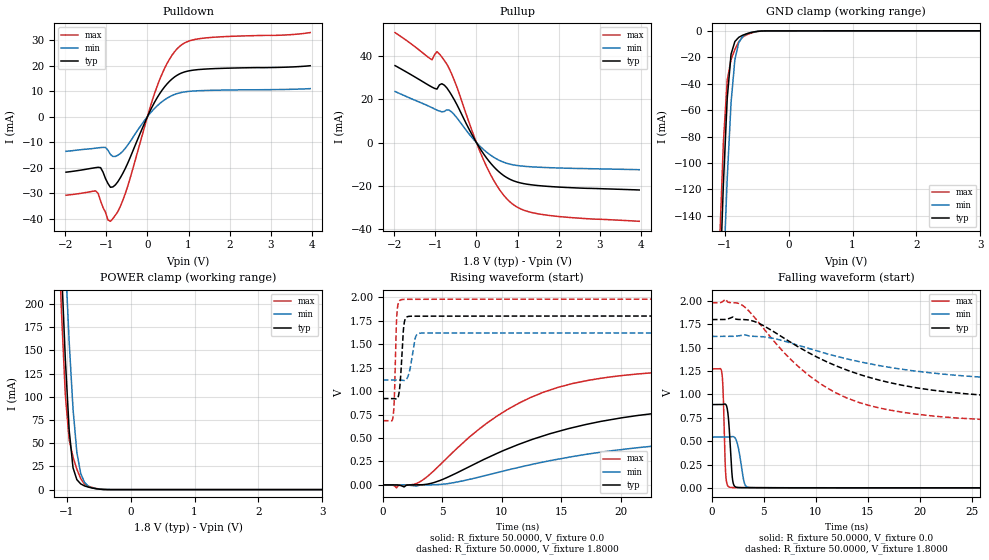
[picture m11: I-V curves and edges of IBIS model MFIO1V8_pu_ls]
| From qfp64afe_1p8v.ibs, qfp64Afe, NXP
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[Model] MFIO1V8_pu_ls
|   Model MFIO1V8_pu_ls
| This model was characterised for following simulation conditions:
| External (pad) voltage:
|   - Typ: 1.8V,   - Min: 1.62V,   - Max: 1.98V
| Library cells for typ/min/max conditions are connected as defined below:
|  IO - External Pad
|  A - Core Input
|  EN - Output Buffer Enable
|  BOOST - vdde
|  EHS - gnd
|  ENZI - vdd
|  EPD - gnd
|  EPUN - gnd
|  ZI - NC
|  ZIF - NC
|  gnd - gnd
|  gnde - gnde
|  vdd - vdd
|  vdde - vdde
| All other pins connected to ground
Model_type I/O
Polarity   Non-Inverting
Enable   Active-Low
Vinl =   0.5400V
Vinh =   1.2600V
Vmeas =  0.9000V
Cref =   0.0F
Rref =   100.0000
Vref =   0.0V
C_comp   1.5959pF   1.5126pF   1.6704pF
|C_comp_pullup   0.7872pF   0.8189pF   0.7436pF
|C_comp_pulldown   0.5957pF   0.6344pF   0.5599pF
[Model Spec]
| variable   typ   min   max
Vinh   0.5400V   0.4860V   0.5940V
Vinl   1.2600V   1.1340V   1.3860V
Vmeas   0.9000V   0.8100V   0.9900V
[Temperature Range]   25.0000   0.1250k   -40.0000
[Voltage Range]   1.8000V   1.6200V   1.9800V
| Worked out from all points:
|   slope of the pulldown table from 0 to 0.27 V, typ, clamps not added: 32.6 ohm
|   slope of the pullup table from 0 to 0.27 V, typ, clamps not added: 34.8 ohm
|   GND clamp passes 1 mA (typ) near -0.56 V on its own axis
|   POWER clamp passes 1 mA (typ) near -0.54 V on its own axis
|   rising waveform, R_fixture 50.0000, V_fixture 0.0: 20-80 % time 12.9ns typ, 15.7ns min, 9.09ns max; typ from 0.001 V to 0.891 V
|   rising waveform, R_fixture 50.0000, V_fixture 1.8000: 20-80 % time 250ps typ, 393ps min, 168ps max; typ from 0.921 V to 1.8 V
|   falling waveform, R_fixture 50.0000, V_fixture 0.0: 20-80 % time 296ps typ, 476ps min, 197ps max; typ from 0.891 V to 0.001 V
|   falling waveform, R_fixture 50.0000, V_fixture 1.8000: 20-80 % time 11.7ns typ, 13.6ns min, 8.56ns max; typ from 1.8 V to 0.921 V
[Pulldown]
|Voltage   I(typ)   I(min)   I(max)
-1.98V    -21.74mA   -13.58mA   -30.76mA
-1.26V    -19.96mA   -12.33mA   -29.04mA
-1.14V    -19.96mA   -12.1mA    -33mA
-960mV    -26.19mA   -13.15mA   -40.44mA
-840mV    -27.51mA   -15.58mA   -39.92mA
-540mV    -20.34mA   -12.41mA   -30.2mA
60mV      2.086mA    1.197mA    3.341mA
300mV     9.043mA    5.145mA    14.58mA
540mV     13.88mA    7.813mA    22.59mA
840mV     17.16mA    9.517mA    28.23mA
1.44V     18.67mA    10.27mA    30.87mA
3.96V     19.95mA    10.98mA    32.93mA
[Pullup]
|Voltage   I(typ)   I(min)   I(max)
-1.98V    35.7mA     23.68mA    51.03mA
-1.08V    25.71mA    16.17mA    38.42mA
-960mV    24.81mA    15.04mA    42.18mA
-840mV    27.29mA    14.27mA    39.65mA
-720mV    25.36mA    15.21mA    36.42mA
-540mV    19.88mA    12.94mA    28.95mA
-60mV     2.002mA    1.263mA    3.041mA
240mV     -7.02mA    -4.333mA   -10.88mA
600mV     -14.41mA   -8.644mA   -22.88mA
900mV     -17.74mA   -10.36mA   -28.83mA
1.74V     -20.33mA   -11.62mA   -33.75mA
3.96V     -22mA      -12.58mA   -36.53mA
[GND_clamp]
|Voltage   I(typ)   I(min)   I(max)
-1.98V    -1.781A    -1.801A    -1.77A
-1.08V    -200.2mA   -270.3mA   -162.2mA
-1.02V    -116mA     -186.3mA   -84.54mA
-960mV    -51.3mA    -111.9mA   -37.4mA
-900mV    -17.69mA   -54.47mA   -21.74mA
-840mV    -8.055mA   -21.72mA   -14.12mA
-780mV    -4.959mA   -8.992mA   -8.359mA
-720mV    -3.374mA   -4.47mA    -4.799mA
-600mV    -1.439mA   -1.366mA   -1.942mA
-480mV    -366uA     -375.1uA   -469.4uA
-360mV    -62.42uA   -67.25uA   -76.06uA
3.96V     0A         0A         0A
[POWER_clamp]
|Voltage   I(typ)   I(min)   I(max)
-1.98V    2.119A     2.147A     2.105A
-1.14V    349.2mA    450mA      300.5mA
-1.08V    239.1mA    345.9mA    191.2mA
-1.02V    140.4mA    247.8mA    101.6mA
-960mV    64.04mA    159.3mA    53.84mA
-900mV    23.56mA    87.21mA    35.07mA
-840mV    10.75mA    40.17mA    22.03mA
-780mV    6.182mA    17.48mA    11.88mA
-720mV    3.977mA    7.724mA    5.963mA
-600mV    1.704mA    1.818mA    2.322mA
-360mV    31.78uA    68.22uA    27.15uA
3.96V     0A         0A         0A
[Ramp]
| variable   typ   min   max
dV/dt_r  0.5342/12.9472n   0.3254/15.7052n   0.7632/9.0881n
dV/dt_f  0.5274/11.7431n   0.3009/13.6080n   0.7767/8.5548n
R_load = 50.0000
[Rising Waveform]
R_fixture= 50.0000
V_fixture= 0.0
V_fixture_min= 0.0
V_fixture_max= 0.0
|time   V(typ)   V(min)   V(max)
0s        636.5uV    684uV      594.3uV
1.143ns   588.1uV    702uV      -30.91mV
3.203ns   1.63mV     -537.3uV   39.42mV
4.956ns   55.11mV    6.837mV    232.7mV
8.014ns   241.9mV    81.4mV     587.6mV
12.33ns   474.1mV    212.9mV    926.3mV
15.97ns   611.4mV    303mV      1.081V
21.24ns   736.7mV    394.5mV    1.18V
40.28ns   869.7mV    518mV      1.262V
100ns     890.9mV    543.1mV    1.273V
[Rising Waveform]
R_fixture= 50.0000
V_fixture= 1.8000
V_fixture_min= 1.6200
V_fixture_max= 1.9800
|time   V(typ)   V(min)   V(max)
0s        920.9mV    1.118V     685.4mV
847.9ps   921.1mV    1.118V     718.1mV
969.6ps   919.2mV    1.119V     934.2mV
1.204ns   918.4mV    1.119V     1.857V
1.441ns   1.063V     1.117V     1.968V
1.682ns   1.563V     1.114V     1.977V
1.952ns   1.783V     1.121V     1.978V
2.739ns   1.798V     1.572V     1.978V
3.266ns   1.798V     1.618V     1.978V
100ns     1.8V       1.62V      1.98V
[Falling Waveform]
R_fixture= 50.0000
V_fixture= 0.0
V_fixture_min= 0.0
V_fixture_max= 0.0
|time   V(typ)   V(min)   V(max)
0s        891mV      543.2mV    1.273V
954.2ps   891.2mV    543.2mV    1.237V
1.08ns    893.2mV    543.2mV    1.041V
1.347ns   891.4mV    543mV      127mV
1.579ns   763.2mV    544mV      15.76mV
1.811ns   371.8mV    547.1mV    5.267mV
2.131ns   27.06mV    545.1mV    3.544mV
3.155ns   2.666mV    43.29mV    3.519mV
3.779ns   2.782mV    2.922mV    2.864mV
100ns     636.6uV    684.1uV    594.3uV
[Falling Waveform]
R_fixture= 50.0000
V_fixture= 1.8000
V_fixture_min= 1.6200
V_fixture_max= 1.9800
|time   V(typ)   V(min)   V(max)
0s        1.8V       1.62V      1.98V
1.307ns   1.801V     1.62V      2.019V
3.054ns   1.8V       1.635V     1.944V
4.714ns   1.75V      1.618V     1.741V
7.87ns    1.538V     1.54V      1.344V
11.77ns   1.314V     1.413V     1.025V
15.21ns   1.18V      1.327V     879.4mV
20.58ns   1.056V     1.236V     776.8mV
39.7ns    937.8mV    1.133V     694.9mV
100ns     921mV      1.118V     685.4mV
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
